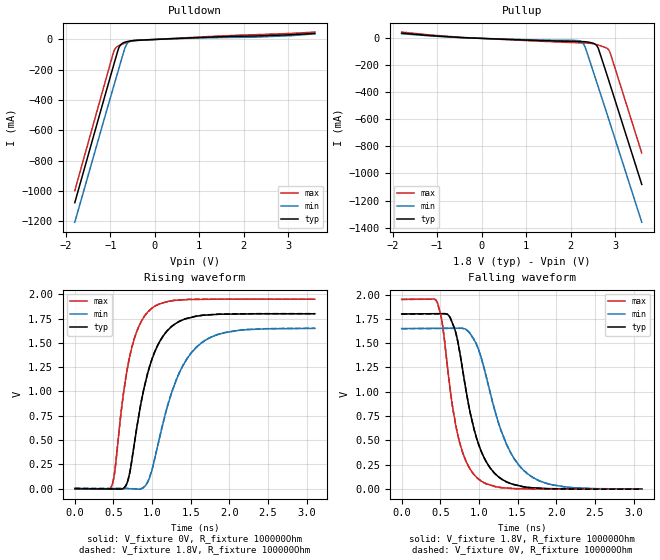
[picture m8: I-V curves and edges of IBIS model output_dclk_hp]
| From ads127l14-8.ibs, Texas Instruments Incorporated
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|   output_dclk_hp Model
[Model]   output_dclk_hp
Model_type   Output
Polarity   Non-Inverting
Vmeas = 0.9
Vref = 0
Cref = 2pF
Rref = 100000
|   typ   min   max
C_comp   0.591pF   0.619pF   0.582pF
[Voltage Range]   1.8   1.65   1.95
[Temperature Range]   27   125   -40
[Pullup Reference]   1.8   1.65   1.95
[Pulldown Reference]   0   0   0
[Power Clamp Reference]   1.8   1.65   1.95
[GND Clamp Reference]   0   0   0
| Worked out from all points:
|   slope of the pulldown table from 0 to 0.27 V, typ, clamps not added: 75.1 ohm
|   slope of the pullup table from 0 to 0.27 V, typ, clamps not added: 77.9 ohm
|   falling waveform, V_fixture 1.8V, R_fixture 100000Ohm: 20-80 % time 301ps typ, 403ps min, 234ps max; typ from 1.8 V to 0.001 V
|   rising waveform, V_fixture 0V, R_fixture 100000Ohm: 20-80 % time 301ps typ, 399ps min, 230ps max; typ from 0 V to 1.8 V
|   rising waveform, V_fixture 1.8V, R_fixture 100000Ohm: 20-80 % time 301ps typ, 399ps min, 230ps max; typ from 0.001 V to 1.8 V
|   falling waveform, V_fixture 0V, R_fixture 100000Ohm: 20-80 % time 301ps typ, 403ps min, 234ps max; typ from 1.8 V to 0 V
[Pulldown]
|   Voltage   I(typ)   I(min)   I(max)
-1.8V     -1.076A    -1.205A    -996.8mA
-1.071V   -318.7mA   -456.5mA   -231.6mA
-914.4mV  -157.8mA   -298mA     -73.32mA
-871.2mV  -113.9mA   -254.3mA   -52.69mA
-817.2mV  -61.31mA   -199.9mA   -42.34mA
-774mV    -36.01mA   -156.4mA   -36.62mA
-671.4mV  -17.82mA   -56.06mA   -24.24mA
-639mV    -15.19mA   -34.5mA    -20.76mA
-590.4mV  -11.95mA   -16.64mA   -16.16mA
-369mV    -4.99mA    -4.049mA   -6.211mA
2.261V    22.91mA    15.45mA    31.55mA
3.6V      39.87mA    36.82mA    48.69mA
[Pullup]
|   Voltage   I(typ)   I(min)   I(max)
-1.8V     38.99mA    34.48mA    46.68mA
-444.6mV  5.876mA    4.778mA    7.406mA
2.093V    -22.41mA   -15.06mA   -31.52mA
2.25V     -23.54mA   -26.51mA   -33.34mA
2.326V    -25.04mA   -64.27mA   -34.2mA
2.531V    -38.35mA   -267.6mA   -40.98mA
2.585V    -51.7mA    -322mA     -45.28mA
2.628V    -78.38mA   -365.6mA   -49.42mA
2.812V    -263.7mA   -551.7mA   -71.81mA
2.871V    -324.9mA   -612.2mA   -93.47mA
2.984V    -441.9mA   -728.1mA   -204.6mA
3.6V      -1.081A    -1.36A     -848.4mA
[Ramp]
R_load = 100000
|   typ   min   max
dV/dt_r   1.07917/3.0098e-10   0.989044/3.97748e-10   1.16929/2.30569e-10
dV/dt_f   1.0792/3.00433e-10   0.989082/4.0237e-10   1.1693/2.3414e-10
[Falling Waveform]
V_fixture = 1.8V
V_fixture_min = 1.65V
V_fixture_max = 1.95V
R_fixture = 100000Ohm
C_fixture = 0F
|   Time   V(typ)   V(min)   V(max)
0s        1.8V       1.65V      1.95V
458.4ps   1.803V     1.652V     1.923V
527.4ps   1.803V     1.653V     1.696V
620ps     1.773V     1.653V     1.074V
718.5ps   1.547V     1.654V     585.3mV
876.2ps   827.1mV    1.609V     219.4mV
991.7ps   470.8mV    1.442V     105.6mV
1.359ns   74.72mV    457.8mV    11.99mV
1.636ns   18.95mV    154.2mV    3.648mV
3.107ns   1.332mV    1.544mV    1.088mV
[Rising Waveform]
V_fixture = 0V
V_fixture_min = 0V
V_fixture_max = 0V
R_fixture = 100000Ohm
C_fixture = 0F
|   Time   V(typ)   V(min)   V(max)
0s        5.4nV      48.21nV    55.4nV
476.5ps   -3.674mV   279uV      23.91mV
637.4ps   4.768mV    373.2uV    1.02V
718.5ps   192.8mV    -1.124mV   1.386V
859.8ps   892.7mV    -1.085mV   1.719V
991.7ps   1.314V     172.6mV    1.852V
1.255ns   1.668V     991.5mV    1.932V
1.572ns   1.774V     1.453V     1.946V
2.121ns   1.796V     1.628V     1.949V
3.107ns   1.799V     1.648V     1.949V
[Rising Waveform]
V_fixture = 1.8V
V_fixture_min = 1.65V
V_fixture_max = 1.95V
R_fixture = 100000Ohm
C_fixture = 0F
|   Time   V(typ)   V(min)   V(max)
0s        1.332mV    1.528mV    1.161mV
476.5ps   -2.319mV   1.806mV    25.14mV
632.4ps   3.077mV    1.896mV    994mV
718.5ps   194.5mV    420.9uV    1.388V
859.8ps   894.5mV    557uV      1.72V
991.7ps   1.315V     174.7mV    1.853V
1.255ns   1.67V      993.8mV    1.933V
1.572ns   1.775V     1.455V     1.948V
2.121ns   1.798V     1.63V      1.95V
3.107ns   1.8V       1.65V      1.95V
[Falling Waveform]
|Gnd
V_fixture = 0V
V_fixture_min = 0V
V_fixture_max = 0V
R_fixture = 100000Ohm
C_fixture = 0F
|   Time   V(typ)   V(min)   V(max)
0s        1.799V     1.648V     1.949V
458.4ps   1.802V     1.651V     1.922V
527.4ps   1.802V     1.651V     1.694V
620ps     1.772V     1.652V     1.073V
718.5ps   1.546V     1.652V     583.9mV
876.2ps   825.2mV    1.607V     218.1mV
991.7ps   469.1mV    1.44V      104.4mV
1.359ns   73.32mV    455.7mV    10.83mV
1.636ns   17.6mV     152.4mV    2.486mV
3.107ns   576.9nV    17.2uV     -72.78uV
